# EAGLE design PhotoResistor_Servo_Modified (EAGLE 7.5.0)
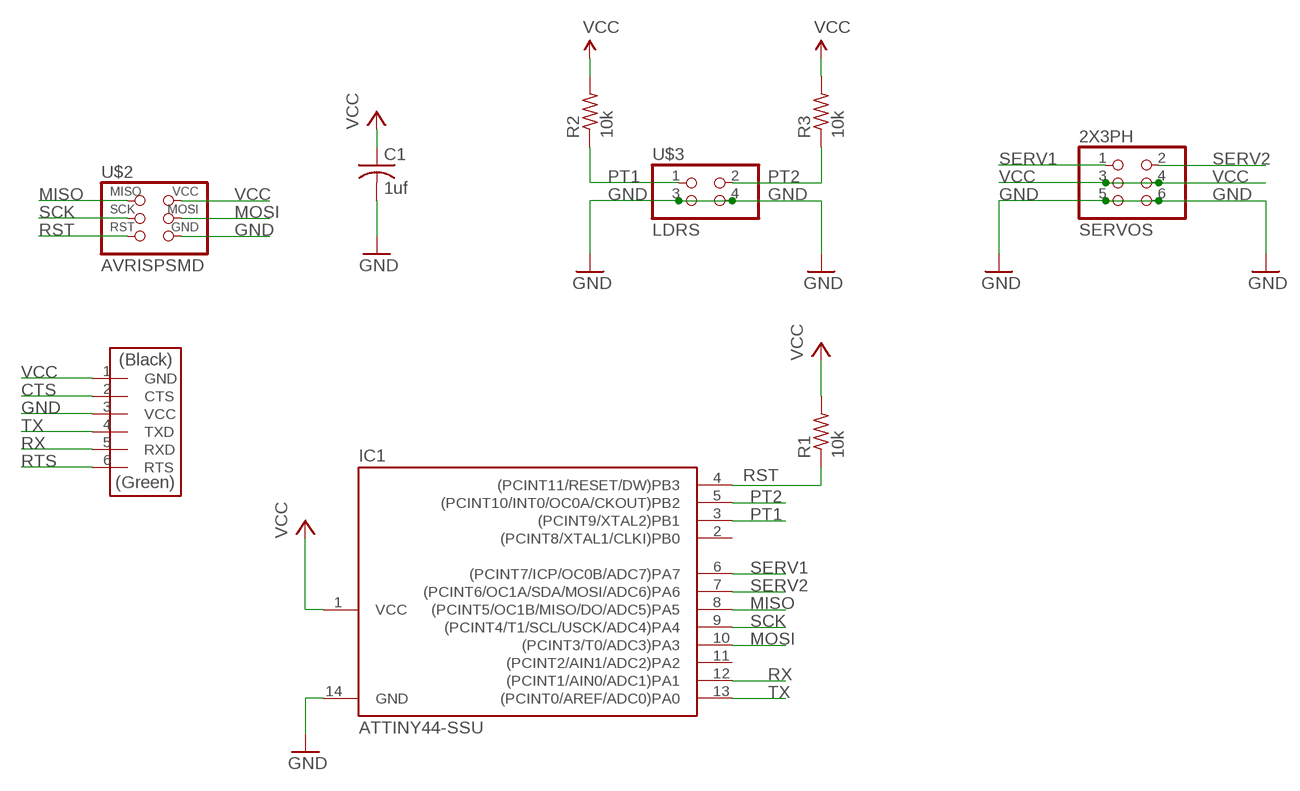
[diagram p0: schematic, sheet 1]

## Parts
2X3PH  SERVOS  PINHD-2X3-SMD  [2X03SMD]
C1  1uf  C-USC1206  [C1206]
IC1  ATTINY44-SSU  [SOIC14]
R1  10k  R-US_R1206  [R1206]
R2  10k  R-US_R1206  [R1206]
R3  10k  RES-US1206  [R1206]
U$2  AVRISPSMD  [2X03SMD]
U$3  LDRS  PINHD-2X2-SMD  [2X02SMD]
U$4  FTDI-SMD-HEADER  [1X06SMD]

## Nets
CTS: U$4.2(CTS)
GND: 2X3PH.5 2X3PH.6 C1.2 IC1.14(GND) U$2.6(GND) U$3.3 U$3.4 U$4.3(VCC)
MISO: IC1.8((PCINT5/OC1B/MISO/DO/ADC5)PA5) U$2.1(MISO)
MOSI: IC1.10((PCINT3/T0/ADC3)PA3) U$2.4(MOSI)
PT1: IC1.3((PCINT9/XTAL2)PB1) R2.1 U$3.1
PT2: IC1.5((PCINT10/INT0/OC0A/CKOUT)PB2) R3.1 U$3.2
RST: IC1.4((PCINT11/RESET/DW)PB3) R1.1 U$2.5(RST)
RTS: U$4.6(RTS)
RX: IC1.12((PCINT1/AIN0/ADC1)PA1) U$4.5(RXD)
SCK: IC1.9((PCINT4/T1/SCL/USCK/ADC4)PA4) U$2.3(SCK)
SERV1: 2X3PH.1 IC1.6((PCINT7/ICP/OC0B/ADC7)PA7)
SERV2: 2X3PH.2 IC1.7((PCINT6/OC1A/SDA/MOSI/ADC6)PA6)
TX: IC1.13((PCINT0/AREF/ADC0)PA0) U$4.4(TXD)
VCC: 2X3PH.3 2X3PH.4 C1.1 IC1.1(VCC) R1.2 R2.2 R3.2 U$2.2(VCC) U$4.1(GND)
Unconnected: IC1.2((PCINT8/XTAL1/CLKI)PB0) IC1.11((PCINT2/AIN1/ADC2)PA2)

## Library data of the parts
2X3PH = fab:PINHD-2X3-SMD: PIN HEADER
C1 = rcl:C-US: CAPACITOR, American symbol
IC1 = fab:ATTINY44
R1 R2 = resistor:R-US_: RESISTOR, American symbol
R3 = fab:RES-US: Resistor (US Symbol)
U$2 = fab:AVRISP
U$3 = fab:PINHD-2X2-SMD
U$4 = fab:FTDI-SMD-HEADER

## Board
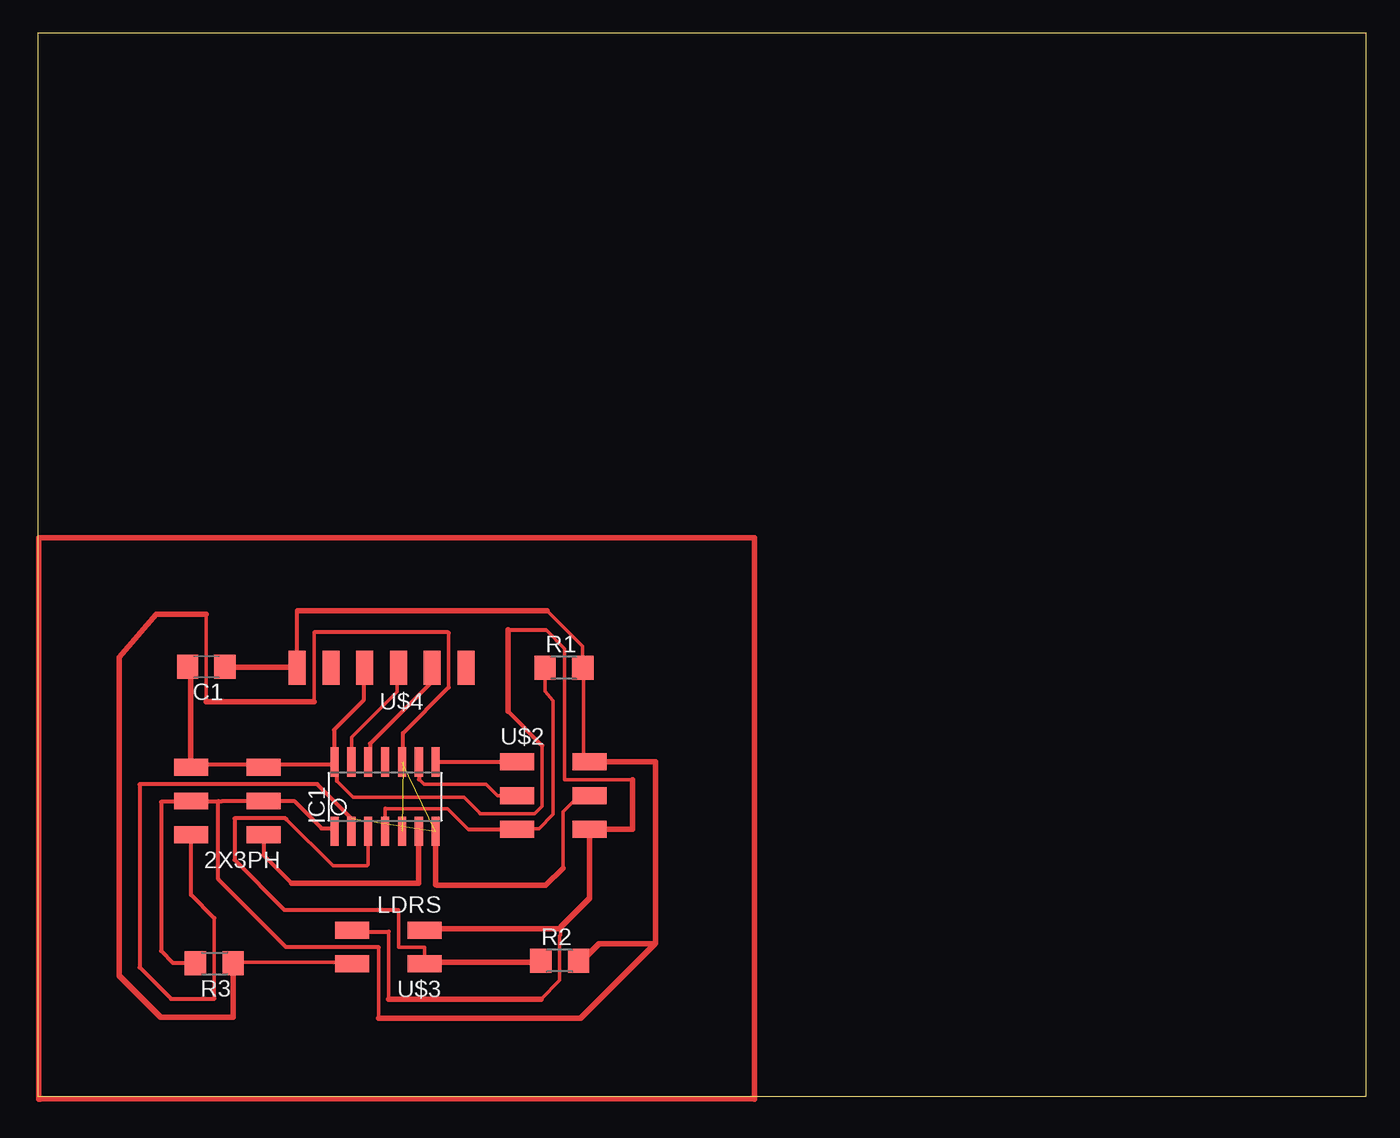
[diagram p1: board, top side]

Size 100 x 80 mm. Coordinates in mm from the lower left corner, seen from the top.
Outline: 0,0 100,0 100,80 0,80 0,0
Copper layers (1*16): Top 0.035mm / dielectric 1.5mm / Bottom 0.035mm
Design rules "default": minimum track width 10mil, minimum drill 24mil, track to track 8mil, track to pad 8mil, pad to pad 8mil, via to via 8mil, smd to smd 8mil, copper to edge 40mil, drill to drill 8mil, minimum pad ring 10mil, minimum via ring 8mil, stop-mask expansion 4mil, vias tented up to drill 0mil, thermal gap 10mil

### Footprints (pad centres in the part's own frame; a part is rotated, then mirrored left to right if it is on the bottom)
2X03SMD = smd 2.54 x 1.27: 1 -2.54,2.54; 2 2.92,2.54; 3 -2.54,0; 4 2.92,0; 5 -2.54,-2.54; 6 2.92,-2.54
C1206 = smd 1.6 x 1.8: 1 -1.4,0; 2 1.4,0
SOIC14 = smd 0.61 x 2.21: 1 -3.81,-2.603; 2 -2.54,-2.603; 3 -1.27,-2.603; 4 0,-2.603; 5 1.27,-2.603; 6 2.54,-2.603; 7 3.81,-2.603; 8 3.81,2.603; 9 2.54,2.603; 10 1.27,2.603; 11 0,2.603; 12 -1.27,2.603; 13 -2.54,2.603; 14 -3.81,2.603
R1206 = smd 1.6 x 1.803: 1 -1.422,0; 2 1.422,0
2X02SMD = smd 2.54 x 1.27: 1 -2.54,1.27; 2 2.92,1.27; 3 -2.54,-1.27; 4 2.92,-1.27
1X06SMD = smd 2.54 x 1.27: 1 0,6.35; 2 0,3.81; 3 0,1.27; 4 0,-1.27; 5 0,-3.81; 6 0,-6.35

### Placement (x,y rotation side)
2X3PH  14.46,22.23 180 top
C1  12.69,32.33 180 top
IC1  26.14,22.55 0 top
R1  39.6,32.25 0 top
R2  39.28,10.22 0 top
R3  13.29,10.01 180 top
U$2  38.61,22.63 0 top
U$3  26.57,11.24 180 top
U$4  25.88,32.25 90 top

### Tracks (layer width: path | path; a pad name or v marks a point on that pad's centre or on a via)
GND
  Top 0.254: 23.59,12.62 U$3.4 | 24.34,12.49 23.71,12.49 U$3.4 | 11.49,32.28 C1.2 | 11.49,24.97 2X3PH.6 11.72,24.97 | 22.24,24.97 IC1.14 | 17.21,24.97 2X3PH.5 16.98,24.97 | 24.52,32.05 U$4.3 | 22.46,25.2 IC1.14 | 24.29,12.39 U$3.4 | 29.32,12.62 U$3.3 | 22.46,24.28 22.46,24.97 IC1.14 | 26.41,12.39 26.41,7.3 | 22.5,23.75 23.75,22.5 32.09,22.5 33.24,21.35 33.24,21.32 33.28,21.28 37.41,21.28 37.97,21.84 37.97,26.4 | 38.24,35.1 39.65,33.69 39.65,33.61 39.64,33.6 39.64,23.82 44.76,23.82 | 37.87,7.3 39.29,8.72 39.29,12.09 39.33,12.13 39.33,12.71
  Top 0.305: 24.52,32.05 24.52,29.79 22.3,27.57 22.3,25.18 IC1.14 | 22.24,24.97 17.2,24.97 2X3PH.5 | 16.98,24.97 11.74,24.97 2X3PH.6 | 24.29,12.39 26.41,12.39 | 39.24,12.62 39.33,12.71 39.39,12.77 | 22.46,24.28 22.5,24.25 22.5,23.75 | 35.4,35.1 38.24,35.1 | 35.4,28.97 37.97,26.4
  Top 0.406: U$3.4 | 11.49,24.97 11.49,32.28 | 26.41,7.3 37.87,7.3 | 29.32,12.62 39.24,12.62 | 35.4,28.97 35.4,35.1 | 44.76,23.82 44.76,20.09 U$2.6 41.53,14.91 39.39,12.77
MISO
  Top 0.254: IC1.8 30.01,25.2 30.03,25.17
  Top 0.305: 30.03,25.17 U$2.1
MOSI  (1 unrouted)
  Top 0.254: 41.53,22.45 U$2.4 | 41.44,22.63 U$2.4 | 41.28,22.63 U$2.4 | 29.93,15.91 30.02,15.82 30.08,15.88 | U$2.4 40.74,22.63 39.53,21.42 39.53,17.18
  Top 0.406: 29.93,19.93 29.93,15.91 | 30.08,15.88 38.23,15.88 39.53,17.18
N$1
  Top 0.406: 0.19,-0.19 53.96,-0.2 53.96,42.05 0.06,42.04 0.06,-0.2 0.19,-0.2 0.19,-0.19
PT1
  Top 0.254: 24.96,19.86 IC1.3 | 37.78,10.11 R2.1 | 29.32,10.11 U$3.1 | 24.75,19.02 24.75,19.94 IC1.3 | 29.09,10.11 U$3.1 | U$3.1 29.11,11.22 27.15,11.22 27.15,14.03 | 18.71,20.87 22.23,17.35 24.78,17.35 24.87,17.44 IC1.3
  Top 0.305: 18.71,20.87 18.71,20.85 18.65,20.91 14.8,20.91 14.8,17.79 18.56,14.03 27.15,14.03
  Top 0.406: 29.32,10.11 37.78,10.11
PT2  (1 unrouted)
  Top 0.254: U$3.2 23.61,10.11 14.92,10.11 R3.1 14.69,9.88 | 30.93,30.77 30.93,34.87 | 20.81,34.91 20.81,29.69 | 12.68,29.69 12.68,35.63 12.67,36.29
  Top 0.305: 27.5,25.2 27.5,27.34 30.93,30.77 | 30.93,34.87 30.89,34.91 20.81,34.91 | 14.7,5.95 14.71,5.94
  Top 0.406: 20.81,29.69 12.68,29.69 | 14.71,5.94 R3.1 | 12.67,36.29 8.9,36.29 6.14,33.06 6.14,9.06 9.25,5.95 14.7,5.95
RST
  Top 0.254: 37.78,32.05 R1.1 38.18,30.48 38.78,29.77 38.78,21.24 37.72,20.13 36.12,20.13 36.1,20.11 36.07,20.14 U$2.5 | 26.16,21.64 26.16,19.95 | 26.18,21.66 30.86,21.66 32.44,20.08 32.45,20.09
  Top 0.305: 26.16,19.95 IC1.4 | 26.16,21.64 26.18,21.66 | 32.45,20.09 U$2.5
  Top 0.406: 37.85,32.17 R1.1
RX
  Top 0.254: 24.98,25.2 IC1.12 | 29.55,32.05 U$4.5
  Top 0.305: 29.55,32.05 29.55,31.09 25.01,26.55 25.01,25.29 IC1.12
SCK
  Top 0.254: 28.7,23.85 29.07,23.48 33.74,23.48 34.59,22.63 U$2.3
  Top 0.305: IC1.9 28.7,25.13 28.7,23.85
SERV1
  Top 0.254: 28.64,19.25 28.64,19.94 IC1.6
  Top 0.305: 28.64,19.95 IC1.6 | 2X3PH.1 17,18.15 19.11,16.04
  Top 0.406: 19.11,16.04 28.67,16.04 IC1.6
SERV2  (1 unrouted)
  Top 0.254: 13.29,7.37 13.29,13.42
  Top 0.305: 23.6,20.92 21.04,23.48 21.04,23.5 7.69,23.5 7.66,23.47 7.66,9.7 10.03,7.33 13.25,7.33 13.29,7.37 | 11.54,19.19 2X3PH.2 11.54,15.16 13.28,13.42 13.29,13.42
TX
  Top 0.254: IC1.13 23.61,25.2 23.61,27.02 27.04,30.45 27.04,32.05 U$4.4
  Top 0.406: 23.59,25.16 IC1.13
VCC
  Top 0.254: 17.66,22.22 17.21,22.22 2X3PH.3 16.98,22.22 | 22.24,20.16 IC1.1 | 11.72,10.11 R3.2 | 11.49,22.22 2X3PH.4 11.72,22.22 | 14.24,32.28 C1.1 | 19.49,32.28 U$4.1 19.72,32.28 19.72,32.97 | 40.75,10.34 R2.2 40.75,10.11 | 41.21,32.28 R1.2 | 25.67,11.22 25.67,5.92 | R1.2 41.08,32.19 41.08,25.17 U$2.2 | 19.53,36.48 19.57,36.48 19.57,36.56 | 38.34,36.56 41.02,33.88 R1.2 | 46.45,11.47 46.5,11.53
  Top 0.305: 41.04,32.27 R1.2 | 11.49,22.22 11.49,22.17 9.27,22.17 9.27,10.94 10.17,10.04 11.84,10.04 R3.2 | 11.72,22.22 13.58,22.22 | 13.58,22.22 13.89,22.22 | 2X3PH.3 16.98,22.22 13.89,22.22 | 13.89,22.22 13.88,22.21 | R2.2 40.84,10.08 40.84,10.13 | 17.66,22.22 17.66,22.23 19.29,22.23 21.36,20.16 22.12,20.16 IC1.1 | 25.67,5.92 25.67,5.87 | 25.67,11.22 25.65,11.24 18.68,11.24 13.58,16.34 13.58,22.22 | U$4.1 19.53,36.48
  Top 0.406: 19.49,32.28 14.24,32.28 | 25.67,5.87 40.84,5.87 46.45,11.47 42.23,11.47 40.84,10.08 | 19.57,36.56 38.34,36.56 | 46.5,11.53 46.5,25.17 U$2.2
